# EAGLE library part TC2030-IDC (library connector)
The TC2030-IDC is our "Legged" 6-pin Plug-of-Nailstm Cable fitted with a 6-pin 0.1" pitch ribbon connector.
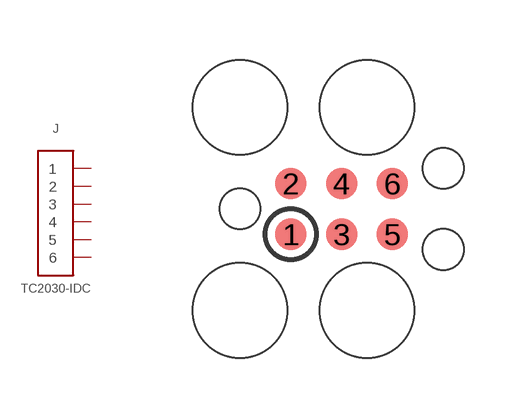
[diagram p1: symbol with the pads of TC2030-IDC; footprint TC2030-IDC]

Designator prefix J

## TC2030-IDC (TAGCONNECT: TC2030-IDC)  [TC2030-IDC]
1  1
2  2
3  3
4  4
5  5
6  6

## Footprint TC2030-IDC (pad centres in mm)
Tag Connect TC2030-IDC
smd 0.787 x 0.787: 1 -1.27,-0.635; 2 -1.27,0.635; 3 0,-0.635; 4 0,0.635; 5 1.27,-0.635; 6 1.27,0.635
hole 2.375 at -2.54,2.54
hole 2.375 at 0.635,2.54
hole 2.375 at 0.635,-2.54
hole 2.375 at -2.54,-2.54
hole 1.016 at -2.54,0
hole 1.016 at 2.54,1.016
hole 1.016 at 2.54,-1.016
